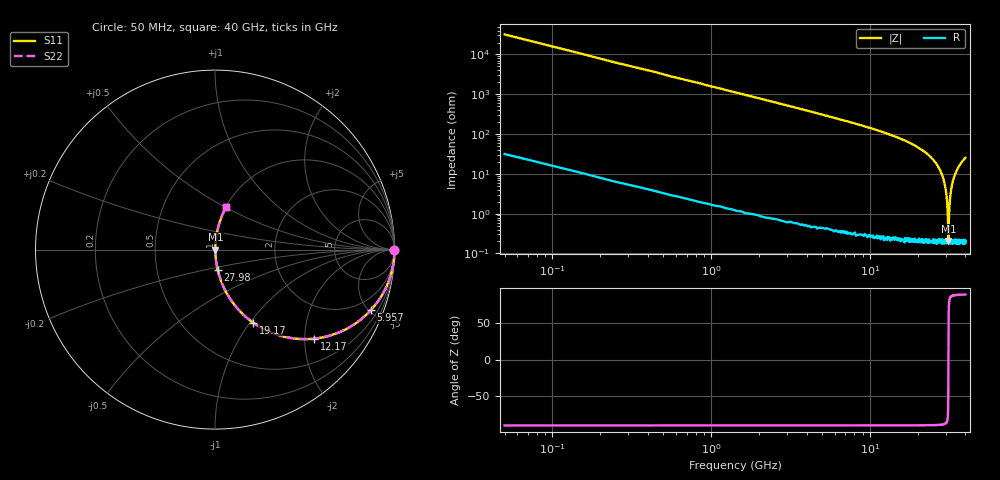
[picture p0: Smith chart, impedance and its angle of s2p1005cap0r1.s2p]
!	AVX	Thin	Film	Operation
!	Date:	March 2012
!	Description: Ultra-Miniature 01005 Size ACCU - P® Thin Film RF / Microwave Capacitor
!	Part Number:  C005YJ0R1ABSTR
!	Serial	Measurements
# MHZ S MA R 50
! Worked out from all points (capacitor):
!   400 points, 50 MHz to 40 GHz, reference 50 ohm
!   read as one part in series: C = 99.9 fF near 250.3 MHz
!   lowest |Z| = 207 mohm at 31.29 GHz (marker M1)
!   series resonance near 31.27 GHz, so ESL is about 260 pH
!   S11 on the Smith chart (normalised r, x): 50 MHz: open; 5.957 GHz: 1.00, -5.15; 12.17 GHz: 1.01, -2.22; 19.17 GHz: 1.00, -1.04; 27.98 GHz: 1.00, -0.23; 40 GHz: 1.00, +0.51
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50  1 -0.2  0.003142 89.8  0.003142 89.8  1 -0.2
150.125  1 -0.5  0.009432 89.4  0.009432 89.4  1 -0.5
350.376  1 -1.3  0.022 88.7  0.022 88.7  1 -1.3
1251.504  0.997 -4.5  0.079 85.4  0.079 85.4  0.997 -4.5
2953.634  0.983 -10.6  0.184 79.3  0.184 79.3  0.983 -10.6
5957.393  0.932 -21.2  0.362 68.7  0.362 68.7  0.932 -21.2
6758.396  0.913 -24.0  0.407 65.9  0.407 65.9  0.913 -24.0
12165.16  0.742 -42.0  0.668 47.9  0.668 47.9  0.742 -42.0
13366.67  0.697 -45.7  0.716 44.2  0.716 44.2  0.697 -45.7
19173.94  0.459 -62.4  0.886 27.3  0.886 27.3  0.459 -62.4
20075.06  0.422 -64.8  0.905 24.9  0.905 24.9  0.422 -64.8
26783.46  0.156 -80.3  0.986 9.0  0.986 9.0  0.156 -80.3
27984.96  0.112 -82.5  0.992 6.5  0.992 6.5  0.112 -82.5
29486.84  0.06 -84.7  0.996 3.4  0.996 3.4  0.06 -84.7
30488.1  0.026 -84.1  0.998 1.5  0.998 1.5  0.026 -84.1
30988.72  0.009489 -77.3  0.998 0.5  0.998 0.5  0.009489 -77.3
31289.1  0.002061 14.6  0.998 -0.0  0.998 -0.0  0.002061 14.6
31489.35  0.00728 73.7  0.998 -0.4  0.998 -0.4  0.00728 73.7
31789.72  0.017 82.2  0.998 -1.0  0.998 -1.0  0.017 82.2
33391.73  0.067 84.5  0.996 -3.8  0.996 -3.8  0.067 84.5
36095.11  0.145 80.9  0.988 -8.3  0.988 -8.3  0.145 80.9
40000  0.245 75.4  0.968 -14.2  0.968 -14.2  0.245 75.4
